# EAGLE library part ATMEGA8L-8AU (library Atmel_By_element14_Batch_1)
8-bit with 8KBytes In-System Programmable Flash
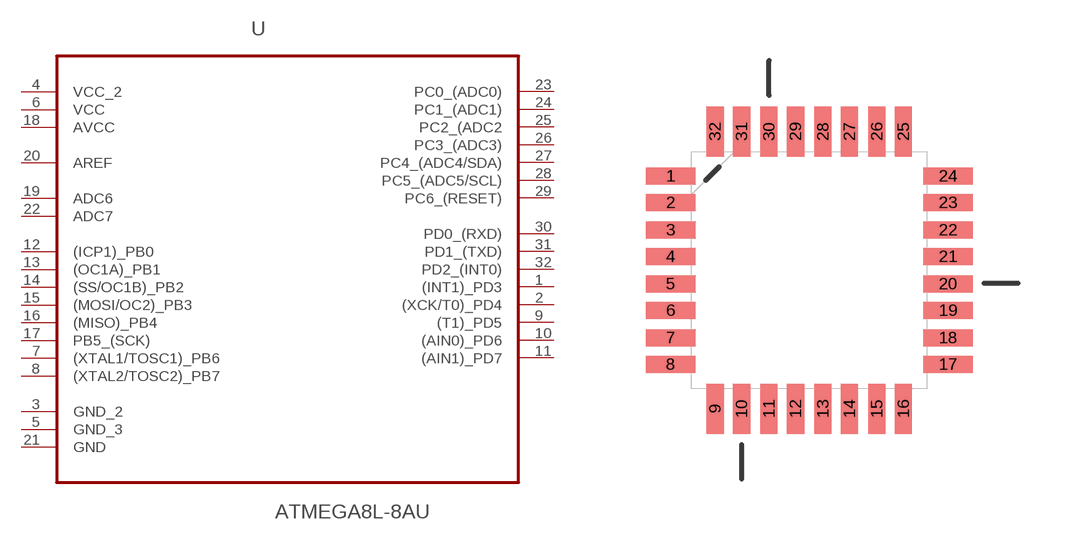
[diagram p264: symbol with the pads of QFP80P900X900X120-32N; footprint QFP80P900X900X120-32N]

Designator prefix U

## ATMEGA8L-8AU (MPN: ATMEGA8L-8AU; OC_FARNELL: 9171525; OC_NEWARK: 68T3210; PACKAGE: QFP-32; SUPPLIER: Atmel)  [QFP80P900X900X120-32N]
1  (INT1)_PD3
2  (XCK/T0)_PD4
3  GND_2  pas
4  VCC_2  pwr
5  GND_3  pas
6  VCC  pwr
7  (XTAL1/TOSC1)_PB6  in
8  (XTAL2/TOSC2)_PB7  out
9  (T1)_PD5
10  (AIN0)_PD6
11  (AIN1)_PD7
12  (ICP1)_PB0
13  (OC1A)_PB1
14  (SS/OC1B)_PB2
15  (MOSI/OC2)_PB3
16  (MISO)_PB4
17  PB5_(SCK)
18  AVCC  pwr
19  ADC6  in
20  AREF  in
21  GND  pas
22  ADC7  in
23  PC0_(ADC0)
24  PC1_(ADC1)
25  PC2_(ADC2
26  PC3_(ADC3)
27  PC4_(ADC4/SDA)
28  PC5_(ADC5/SCL)
29  PC6_(RESET)
30  PD0_(RXD)
31  PD1_(TXD)
32  PD2_(INT0)

## Footprint QFP80P900X900X120-32N (pad centres in mm)
smd 1.473 x 0.508: 1 -4.115,2.794; 2 -4.115,2.007; 3 -4.115,1.194; 4 -4.115,0.406; 5 -4.115,-0.406; 6 -4.115,-1.194; 7 -4.115,-2.007; 8 -4.115,-2.794; 17 4.115,-2.794; 18 4.115,-2.007; 19 4.115,-1.194; 20 4.115,-0.406; 21 4.115,0.406; 22 4.115,1.194; 23 4.115,2.007; 24 4.115,2.794
smd 0.508 x 1.473: 9 -2.794,-4.115; 10 -2.007,-4.115; 11 -1.194,-4.115; 12 -0.406,-4.115; 13 0.406,-4.115; 14 1.194,-4.115; 15 2.007,-4.115; 16 2.794,-4.115; 25 2.794,4.115; 26 2.007,4.115; 27 1.194,4.115; 28 0.406,4.115; 29 -0.406,4.115; 30 -1.194,4.115; 31 -2.007,4.115; 32 -2.794,4.115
